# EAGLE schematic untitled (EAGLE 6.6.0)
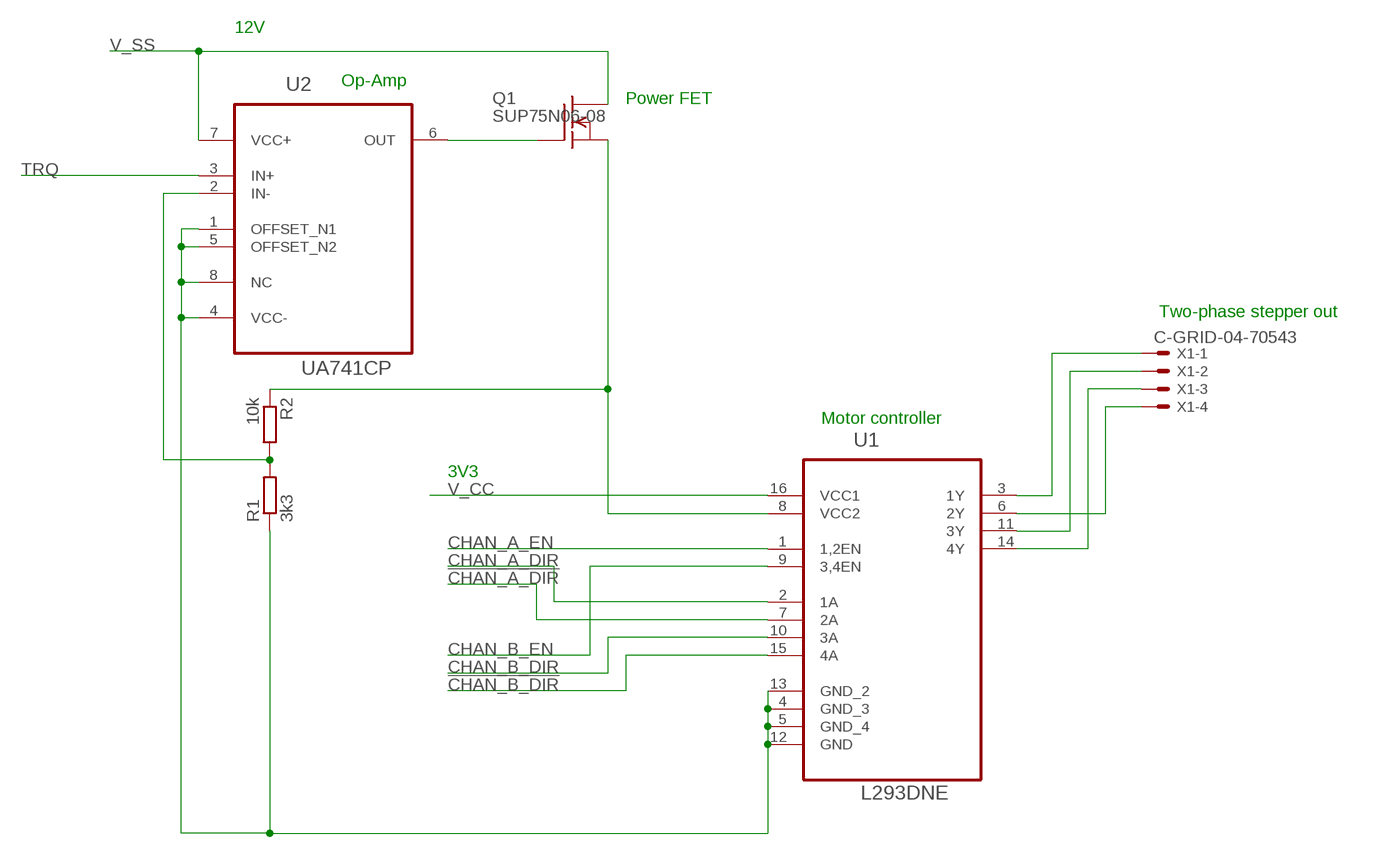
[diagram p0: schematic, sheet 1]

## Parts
Q1  SUP75N06-08  [TO220]
R1  3k3  R-EU_0204/7  [0204/7]
R2  10k  R-EU_0204/7  [0204/7]
U1  L293DNE  [DIP254P762X508-16]
U2  UA741CP  [DIP254P762X508-8]
X1  C-GRID-04-70543  [70543-04]

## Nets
!CHAN_A_DIR: U1.7(2A)
!CHAN_B_DIR: U1.15(4A)
CHAN_A_DIR: U1.2(1A)
CHAN_A_EN: U1.1(1,2EN)
CHAN_B_DIR: U1.10(3A)
CHAN_B_EN: U1.9(3,4EN)
GND: R1.1 U1.4(GND_3) U1.5(GND_4) U1.12(GND) U1.13(GND_2) U2.1(OFFSET_N1) U2.4(VCC-) U2.5(OFFSET_N2) U2.8(NC)
N$1: Q1.3(S) R2.1 U1.8(VCC2)
N$2: Q1.1(G) U2.6(OUT)
N$4: R1.2 R2.2 U2.2(IN-)
N$5: U1.3(1Y) X1.1
N$6: U1.6(2Y) X1.4
N$7: U1.11(3Y) X1.2
N$8: U1.14(4Y) X1.3
TRQ: U2.3(IN+)
V_CC: U1.16(VCC1)
V_SS: Q1.2(D) U2.7(VCC+)

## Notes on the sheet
- 12V
- Op-Amp
- Power FET
- Two-phase stepper out
- Motor controller
- 3V3

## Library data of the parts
Q1 = transistor-fet:SUP75N06-08: N-Channel Enhancement MOSFET 60V; 75A; 0,008Ohm
R1 R2 = resistor:R-EU_: RESISTOR, European symbol
U1 = Texas Instruments_By_element14_Batch_1:L293DNE: QUADRUPLE HALF-H DRIVERS; MPN: L293DNE; OC_FARNELL: 1470423; OC_NEWARK: 06F9523; PACKAGE: PDIP-16; SUPPLIER: Texas Instruments
U2 = Texas Instruments_By_element14_Batch_1:UA741CP: OPERATIONAL AMPLIFIER; MPN: UA741CP; OC_FARNELL: 1564944; OC_NEWARK: 60K7043; PACKAGE: PDIP; SUPPLIER: Texas Instruments
X1 = con-molex:C-GRID-04: CONNECTOR wire to board 2.54 mm (0.100") pitch header; OC_FARNELL: unknown; OC_NEWARK: unknown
